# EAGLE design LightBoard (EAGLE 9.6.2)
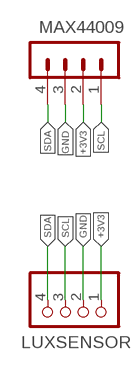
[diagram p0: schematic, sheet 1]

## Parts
LUXSENSOR  PINHD-1X4  [1X04]
MAX44009  B4B-PH-K-S  [B4B-PH-K-S]

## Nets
+3V3: LUXSENSOR.1 MAX44009.2
GND: LUXSENSOR.2 MAX44009.3
SCL: LUXSENSOR.3 MAX44009.1
SDA: LUXSENSOR.4 MAX44009.4

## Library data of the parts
LUXSENSOR = pinhead:PINHD-1X4: PIN HEADER
MAX44009 = con-JSTPH:B4B-PH: JST PH series header 2.00mm pitch disconnectable crimp style connectors, vertical (side entry type), 4 pins

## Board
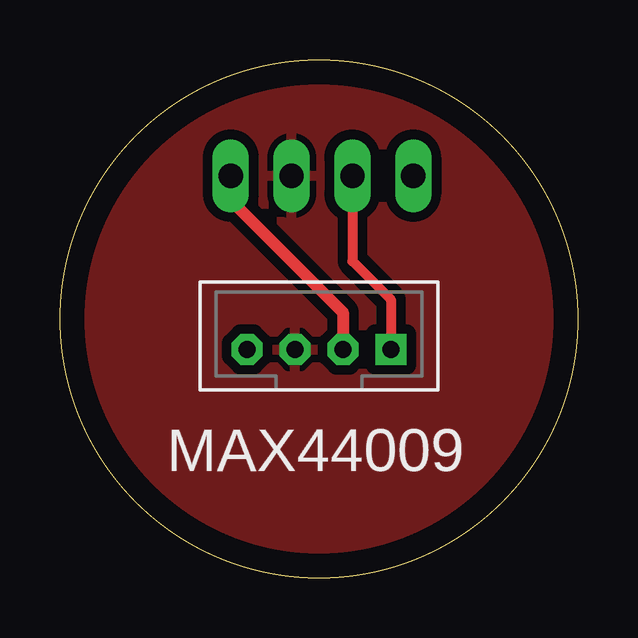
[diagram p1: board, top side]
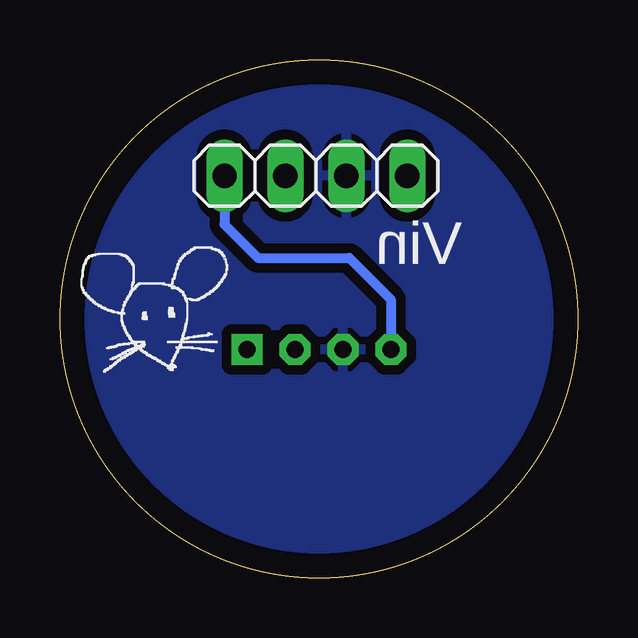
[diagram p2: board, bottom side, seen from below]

Size 21.6 x 21.6 mm. Coordinates in mm from the lower left corner, seen from the top.
Outline: circle at 10.8,10.8 radius 10.8
Copper layers (1*16): Top 0.035mm / dielectric 1.5mm / Bottom 0.035mm
Design rules "default": minimum track width 6mil, minimum drill 0.35mm, track to track 6mil, track to pad 6mil, pad to pad 6mil, via to via 6mil, smd to smd 6mil, copper to edge 40mil, drill to drill 6mil, minimum pad ring 10mil, minimum via ring 8mil, stop-mask expansion 4mil, vias tented up to drill 0mil, thermal gap 10mil

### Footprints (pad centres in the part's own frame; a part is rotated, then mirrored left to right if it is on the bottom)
1X04 = drill 1.016 long: 1 -3.81,0; 2 -1.27,0; 3 1.27,0; 4 3.81,0
B4B-PH-K-S = drill 0.7 pad 1.3 square: 1 3,0 | drill 0.7 pad 1.3 octagon: 2 1,0; 3 -1,0; 4 -3,0

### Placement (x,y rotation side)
LUXSENSOR  10.93,16.77 180 bottom
MAX44009  10.8,9.53 0 top

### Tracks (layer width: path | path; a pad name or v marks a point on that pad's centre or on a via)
+3V3
  Top 0.508: LUXSENSOR.1 7.12,15.75 11.8,11.07 MAX44009.2
GND
  pour Bottom (isolate 0.406): 6.99,22.23 15.88,22.23 22.23,15.88 22.23,5.72 15.88,-0.63 6.99,-0.63 5.72,-0.63 -0.63,5.72 -0.63,15.88 5.72,22.23
  pour Top (isolate 0.406): 5.72,22.23 15.88,22.23 22.23,15.88 22.23,5.72 15.88,-0.63 5.72,-0.63 -0.63,5.72 -0.63,15.88
SCL
  Top 0.406: LUXSENSOR.3 12.2,13.21 13.8,11.61 MAX44009.1
SDA
  Bottom 0.406: LUXSENSOR.4 14.74,14.74 13.34,13.34 9.53,13.34 7.8,11.61 MAX44009.4

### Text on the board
tPlace: MAX44009
bPlace: Vin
